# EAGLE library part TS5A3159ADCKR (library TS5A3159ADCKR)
1 Ohm SPDT Analog Switch 5-V/3.3-V Single Channel 2:1 Multiplexer/Demultiplexer Source: Datasheet
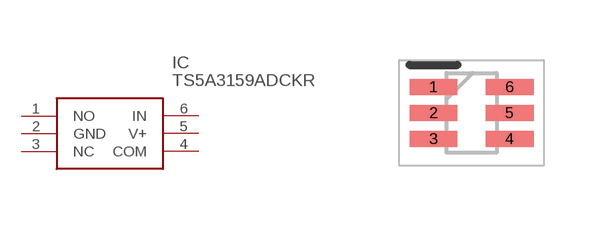
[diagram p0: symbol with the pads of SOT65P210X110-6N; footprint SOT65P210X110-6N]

Designator prefix IC

## TS5A3159ADCKR (Arrow_Part_Number: TS5A3159ADCKR; Arrow_Price-Stock: https://www.arrow.com/en/products/ts5a3159adckr/texas-instruments?utm_currency=USD&region=nac; Description: 1 Ohm SPDT Analog Switch 5-V/3.3-V Single Channel 2:1 Multiplexer/Demultiplexer; Height: 1.1mm; Manufacturer_Name: Texas Instruments; Manufacturer_Part_Number: TS5A3159ADCKR; Mouser_Part_Number: 595-TS5A3159ADCKR; Mouser_Price-Stock: https://www.mouser.co.uk/ProductDetail/Texas-Instruments/TS5A3159ADCKR?qs=0O%2FZFlpUpJWT7PTKGuP8wA%3D%3D)  [SOT65P210X110-6N]
1  NO
2  GND
3  NC  nc
4  COM
5  V+
6  IN

## Footprint SOT65P210X110-6N (pad centres in mm)
DCK-6
smd 1.2 x 0.4: 1 -0.95,0.65; 2 -0.95,0; 3 -0.95,-0.65; 4 0.95,-0.65; 5 0.95,0; 6 0.95,0.65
